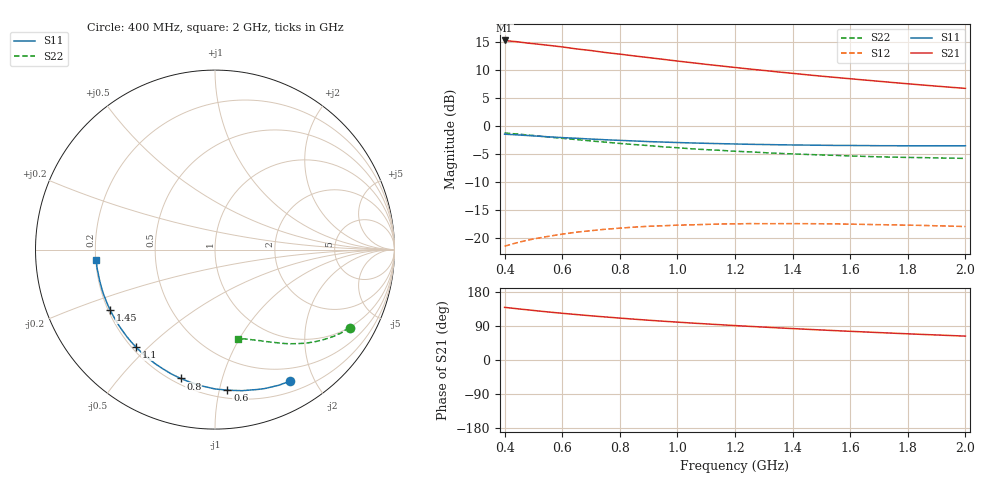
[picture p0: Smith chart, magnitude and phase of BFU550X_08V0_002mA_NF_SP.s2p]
! Filename:  P:\Prog\Test\Noise\ATS_data\Testdata_Net\BFU550X no attenuator noise\BFU550X_APG2013_44_C05_08p0V_002mA_NF_CM01_D.sf
! Date/Time: Fri 26/Jul/2013 14:37:12
! BFU550X_APG2013_44_C05_08p0V_1to10mA_NF_CM01_Bias2_R.sf
! Noise Parameter Data File
! BFU550X_APG2013_44_C05_08p0V_1to10mA_NF_CM01
! Date/time: Wed Jul 24 17:16:38 2013
! VAR V_out= 8.000000
! VAR I_out= 1.995000
! VAR V_in= 0.790100
! VAR I_in= 0.021000
! Device data file deembeded for feedlines and parallel
! Original file: \BFU550X no attenuator noise\BFU550X_APG2013_44_C05_08p0V_002mA_NF_CM01_R.sf
! Feed-files: PR005V01_100713_Feed1.s2p, PR005V01_100713_Feed2.s2p
! Parallel-file: PR005V01_100713_Par.s2p
# MHz S MA R 50
!  Freq-MHz  S11-mag  S11-arg  S21-mag  S21-arg  S12-mag  S12-arg  S22-mag  S22-arg
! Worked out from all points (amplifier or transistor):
!   37 points, 400 MHz to 2 GHz, reference 50 ohm
!   highest |S21| = 15.3 dB at 400 MHz (marker M1)
!   |S21| within 3 dB of that: start of sweep to 889.8 MHz
!   unconditionally stable (mu >= 1): nowhere
!   at 500 MHz: K = 0.16, MSG = 17.4 dB, |S12| = -20.2 dB
!   at 1.1 GHz: K = 0.33, MSG = 14.3 dB, |S12| = -17.6 dB
!   at 2 GHz: K = 0.62, MSG = 12.3 dB, |S12| = -18.0 dB
!   lowest NFmin = 0.54 dB at 460 MHz
!   S11 on the Smith chart (normalised r, x): 400 MHz: 0.33, -1.67; 600 MHz: 0.26, -1.06; 800 MHz: 0.23, -0.74; 1.1 GHz: 0.22, -0.46; 1.45 GHz: 0.21, -0.26; 2 GHz: 0.20, -0.04
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400  0.844 -60.4  5.801 138.9  0.08434 55.2  0.8681 -30.2
440  0.8325 -65.7  5.664 135.6  0.09014 52.6  0.849 -32.5
500  0.8143 -73.2  5.43 130.8  0.09779 48.6  0.8216 -35.9
550  0.8002 -79.2  5.259 126.9  0.1031 45.6  0.7967 -38.5
600  0.7864 -84.9  5.079 123.3  0.108 42.8  0.775 -40.8
650  0.7759 -90.2  4.873 119.9  0.1125 40.2  0.7551 -42.9
700  0.7632 -95.5  4.714 116.6  0.116 37.8  0.734 -45.0
750  0.7528 -100.1  4.526 113.6  0.1195 35.6  0.7163 -46.8
800  0.743 -105.0  4.379 110.6  0.1222 33.4  0.6977 -48.7
850  0.7341 -109.4  4.221 107.7  0.1248 31.4  0.6819 -50.3
900  0.7246 -113.8  4.078 105.0  0.127 29.5  0.6674 -51.8
950  0.7178 -117.8  3.936 102.4  0.1283 27.7  0.6508 -53.5
1050  0.7048 -125.3  3.672 97.5  0.1308 24.5  0.6247 -56.2
1100  0.6993 -128.9  3.548 95.2  0.132 23.1  0.6138 -57.4
1200  0.69 -135.6  3.329 90.9  0.1334 20.3  0.5941 -59.9
1350  0.6791 -144.7  3.035 84.8  0.1341 16.9  0.569 -63.2
1450  0.6743 -150.2  2.864 81.0  0.134 14.8  0.5563 -65.2
1500  0.672 -152.8  2.783 79.2  0.1337 13.9  0.5504 -66.2
1600  0.6692 -157.9  2.64 75.7  0.1326 12.2  0.5396 -68.3
1750  0.6655 -164.8  2.44 70.7  0.1307 10.1  0.5266 -71.1
1850  0.664 -169.1  2.321 67.5  0.1293 8.8  0.5213 -72.8
2000  0.6647 -175.2  2.165 63.0  0.1263 7.5  0.513 -75.5
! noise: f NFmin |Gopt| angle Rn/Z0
400  0.5575  0.5156  26.45  0.1995
460  0.5435  0.4727  38.24  0.1666
600  0.6937  0.4851  46.66  0.1912
800  0.6778  0.4627  63.05  0.1678
1000  0.7588  0.4662  78.79  0.1508
1200  0.8307  0.4765  95.15  0.1308
1400  0.8698  0.4875  109.1  0.1232
1600  0.8492  0.4706  125.8  0.0865
1800  0.9175  0.5457  138.2  0.059
2000  1.004  0.5607  147.6  0.0579
